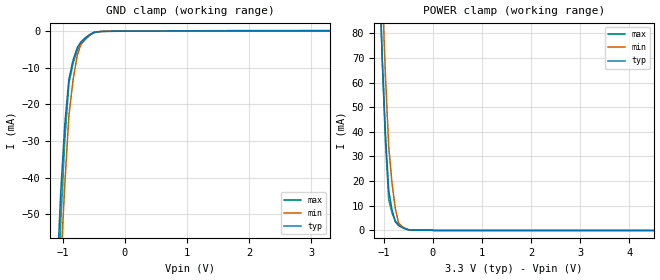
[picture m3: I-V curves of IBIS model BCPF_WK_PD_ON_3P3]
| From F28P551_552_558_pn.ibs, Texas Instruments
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|   Model Cell BCPF_WK_PD_ON_3P3
|BCPF_WK_PD_ON_3P3
[Model]   BCPF_WK_PD_ON_3P3
Model_type   Input
Polarity   Non-Inverting
Vinl =  0.8
Vinh =  2
C_comp   1.21982p   0.982413p   1.3757p
[Model Spec]
Vinl   0.8   0.8   0.8
Vinh   2   2   2
[Temperature Range]   25   155   -40
[Voltage Range]   3.3   2.97   3.63
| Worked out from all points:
|   GND clamp passes 1 mA (typ) near -0.57 V on its own axis
|   POWER clamp passes 1 mA (typ) near -0.61 V on its own axis
| Nom Voltages:
|   BIASFET=3.3, VDD=1.2, VDDS=3.3, VSS=0
| Min Voltages:
|   BIASFET=2.97, VDD=1.08, VDDS=2.97, VSS=0
| Max Voltages:
|   BIASFET=3.63, VDD=1.32, VDDS=3.63, VSS=0
[POWER_clamp]
|   voltage   I(typ)   I(min)   I(max)
-3.3V     1.919A     2.431A     2.069A
-1.1V     109.8mA    140.8mA    113.2mA
-1.033V   70.22mA    98.05mA    69.28mA
-966.7mV  38.97mA    62.35mA    35.68mA
-900mV    16.05mA    33.73mA    12.42mA
-833.3mV  8.293mA    19.1mA     7.096mA
-766.7mV  3.604mA    8.89mA     3.798mA
-700mV    1.979mA    3.094mA    2.529mA
-566.7mV  657.9uA    733.3uA    863uA
-433.3mV  164.3uA    158uA      238.2uA
33.33mV   0A         0A         0A
6.6V      0A         0A         0A
[GND_clamp]
|   voltage   I(typ)   I(min)   I(max)
-3.3V     -1.48A     -1.41A     -2.182A
-1.1V     -69.9mA    -89.89mA   -82.67mA
-1.033V   -44.46mA   -64.18mA   -52.63mA
-966.7mV  -25.51mA   -41.88mA   -29.81mA
-900mV    -13.07mA   -23mA      -14.21mA
-833.3mV  -7.92mA    -13.29mA   -8.777mA
-766.7mV  -4.488mA   -6.652mA   -5.198mA
-700mV    -2.773mA   -3.093mA   -3.475mA
-566.7mV  -923.7uA   -980.4uA   -1.151mA
-500mV    -313.2uA   -412.8uA   -369uA
-300mV    -28uA      -20.59uA   -40.77uA
3.3V      107.2uA    58.9uA     177.9uA
